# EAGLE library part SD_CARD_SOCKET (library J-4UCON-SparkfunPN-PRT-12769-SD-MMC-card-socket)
SD Memory Card Connector (standard "large" size) Push-push normal type, CD enable, WP enable. Here is the connector we sell at SparkFun: SD/MMC Socket (PRT-12769) Datasheet It is used on these SparkFun products: SparkFun SD/MMC Card Breakout (BOB-12941) SD Sniffer (TOL-11468)
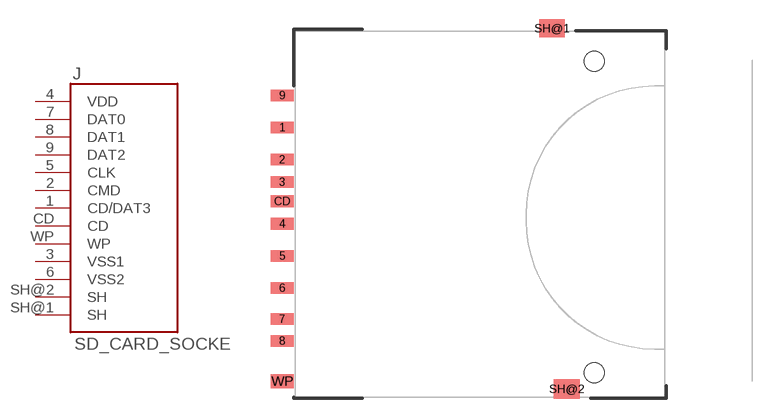
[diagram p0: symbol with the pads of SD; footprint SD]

Designator prefix J

## SD_CARD_SOCKET (PROD_ID: CONN-11976; SF_ID: PRT-12769)  [SD]
1  CD/DAT3
2  CMD
3  VSS1  pwr
4  VDD  pwr
5  CLK
6  VSS2  pwr
7  DAT0
8  DAT1
9  DAT2
CD  CD
SH@1  SH
SH@2  SH
WP  WP

## Footprint SD (pad centres in mm)
SD/MMC Socket Specifications: Pin count:13 Datasheet referenced for footprint Example device(s): SD_CARD_SOCKET
smd 1.8 x 0.9: 1 -1,6.77; 2 -1,4.27; 3 -1,2.52; 4 -1,-0.73; 5 -1,-3.23; 6 -1,-5.73; 7 -1,-8.15; 8 -1,-9.85; 9 -1,9.27; CD -1,1.02
smd 2 x 1.4: SH@1 20,14.496
smd 2 x 1.527: SH@2 21.15,-13.589
smd 1.8 x 1.1: WP -1,-13
hole 1.55 at 23.3,11.94
hole 1.55 at 23.3,-12.32

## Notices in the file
Licensing: Creative Commons ShareAlike 4.0 International - https://creativecommons.org/licenses/by-sa/4.0
